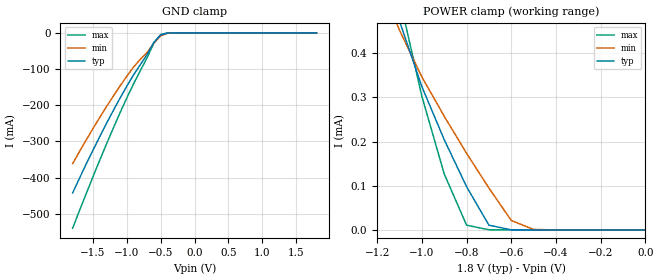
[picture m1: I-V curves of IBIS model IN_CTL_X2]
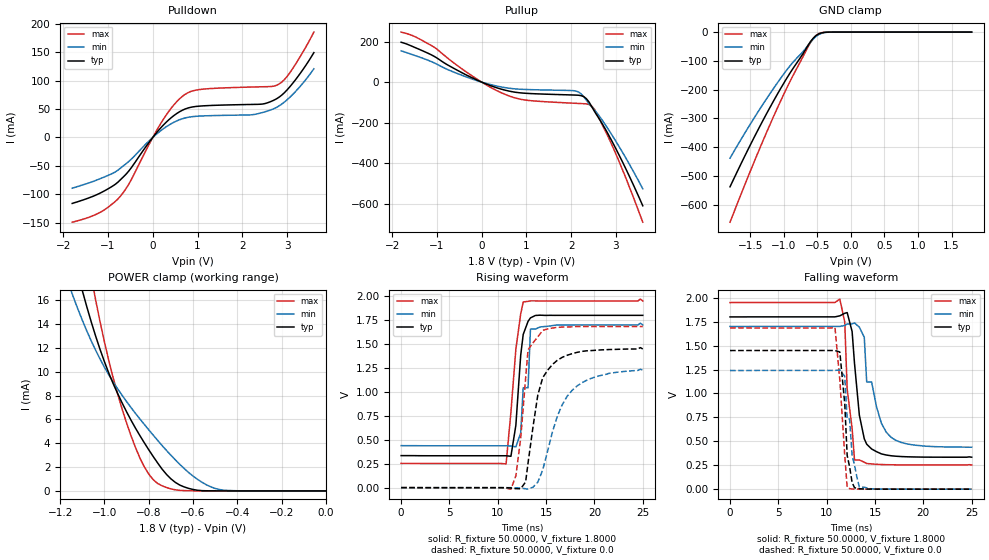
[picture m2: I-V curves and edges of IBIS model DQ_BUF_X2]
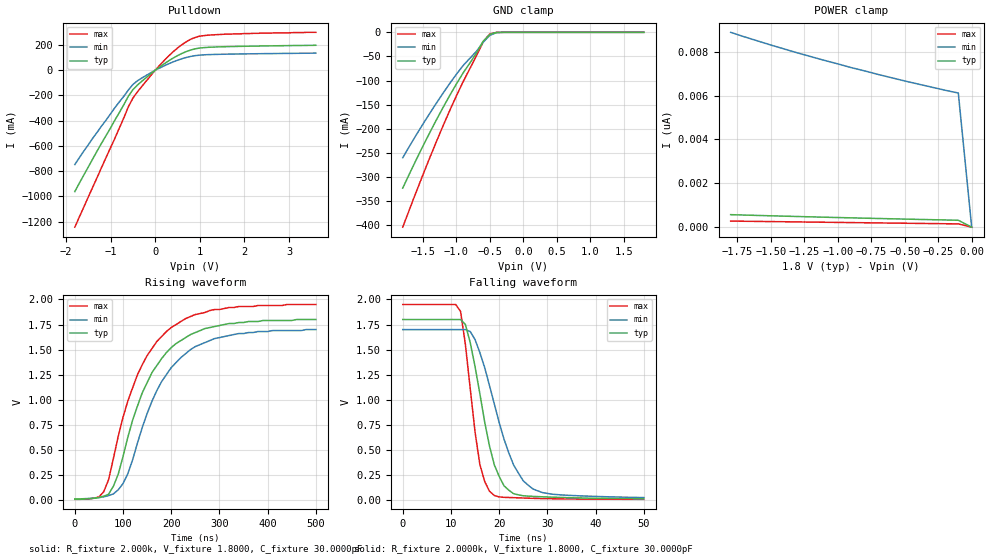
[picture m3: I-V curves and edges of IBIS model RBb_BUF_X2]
| This IBIS file was created by s2ibis3 version 1.1
| North Carolina State University, ERL, 2006
[IBIS ver] 3.2
[File name] s34ms08g2_a_i_18_r2.ibs
[File Rev] 2.0
| Rev1.0 Initial release (X8 LEGACY/ONFI F32 1CE T463ADTX 41086 U785)
| Rev2.0 Update c-comp with measurement
[Date] 1/15/2015
[Source] Cypress IBIS team
[Notes]  Generated IBIS models from SPICE simulations.
|   VIO=1.8V, Temperature Range: Industrial (-40oC to +85oC).
[Disclaimer] THE MODEL LIBRARIES ARE PROVIDED AS IS.
[Copyright] (C) COPYRIGHT 2015
| CYPRESS SEMICONDUCTOR
| ALL RIGHTS RESERVED.
|   Component S34MS08G2 X8 LEGACY/ONFI F32 in VLD063 package
[Component]   S34MS08G2
[Manufacturer]   Cypress
[Package]
| variable   typ   min   max
R_pkg   397.45mOhm   304.71mOhm   533.44mOhm
L_pkg   11.19nH   6.95nH   17.07nH
C_pkg   0.84pF   0.56pF   2.16pF
[Pin]   signal_name   model_name   R_pin   L_pin   C_pin
A1   R   NC
A2   R   NC
A9   R   NC
A10   R   NC
B1   R   NC
B9   R   NC
B10   R   NC
C3   WP   IN_CTL_X2   370.91m   10.638n   2.1652p
C4   ALE   IN_CTL_X2   519.77m   16.877n   0.9751p
C5   VSS   GND
C6   CE#   IN_CTL_X2   533.44m   17.071n   0.9422p
C7   WE#   IN_CTL_X2   393.70m   13.183n   1.0635p
C8   RB#   RBb_BUF_X2  518.54m   16.890n   0.9564p
D3   VCC   NC
D4   RE#   IN_CTL_X2   520.86m   16.856n   0.9647p
D5   CLE   IN_CTL_X2   528.38m   17.047n   0.9436p
D6   R   NC
D7   R   NC
D8   R   NC
E3   R   NC
E4   R   NC
E5   R   NC
E6   R   NC
E7   R   NC
E8   R   NC
F3   R   NC
F4   R   NC
F5   R   NC
F6   R   NC
F7   VSS   NC
F8   R   NC
G3   R   NC
G4   VCC   NC
G5   R   NC
G6   R   NC
G7   R   NC
G8   R   NC
H3   R   NC
H4   IO0   DQ_BUF_X2   310.3m   7.0831n   0.5602p
H5   R   NC
H6   R   NC
H7   R   NC
H8   VCC   POWER
J3   R   NC
J4   IO1   DQ_BUF_X2   313.03m   7.0798n   0.5804p
J5   R   NC
J6   VCC   POWER
J7   IO5   DQ_BUF_X2   330.01m   7.7748n   0.5936p
J8   IO7   DQ_BUF_X2   318.00m   7.1125n   0.5636p
K3   VSS   GND
K4   IO2   DQ_BUF_X2   338.07m   7.8156n   0.5782p
K5   IO3   DQ_BUF_X2   329.94m   7.6927n   0.5743p
K6   IO4   DQ_BUF_X2   331.98m   7.8931n   0.5927p
K7   IO6   DQ_BUF_X2   304.71m   6.9573n   0.5904p
K8   VSS   GND
L1   R   NC
L2   R   NC
L9   R   NC
L10   R   NC
M1   R   NC
M2   R   NC
M9   R   NC
M10   R   NC
| Models and submodels in the file (3): IN_CTL_X2 (Input), DQ_BUF_X2 (I/O), RBb_BUF_X2 (Open_drain)
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|   Model IN_CTL_X2
[Model]   IN_CTL_X2
Model_type   Input
Vinl =   0.3600V
Vinh =   1.4400V
C_comp   6.24pF   5.62pF   8.16pF
[Temperature Range]   25.0000   85.0000   -40.0000
[Voltage Range]   1.8000V   1.7000V   1.9500V
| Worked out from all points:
|   GND clamp passes 1 mA (typ) near -0.41 V on its own axis
|   POWER clamp passes 1 mA (typ) near -1.37 V on its own axis
[GND_clamp]
| voltage   I(typ)   I(min)   I(max)
-1.8V     -442.4mA   -361.4mA   -539.8mA
-1.6V     -362.6mA   -296mA     -444.4mA
-1.4V     -286.6mA   -233.8mA   -351.8mA
-1.1V     -180.2mA   -146.7mA   -220.6mA
-900mV    -115.8mA   -94.34mA   -140.5mA
-700mV    -59.7mA    -54.06mA   -67.86mA
-600mV    -25.92mA   -27.82mA   -28.04mA
-500mV    -5.764mA   -7.906mA   -4.376mA
-400mV    -434.2uA   -908.8uA   -145.6uA
-300mV    -17.2uA    -67.78uA   -1.974nA
1.8V      304.6pA    5.746nA    151.5pA
[POWER_clamp]
| voltage   I(typ)   I(min)   I(max)
-1.8V     2.01mA     1.613mA    2.604mA
-1.1V     472.8uA    452.2uA    525uA
-1V       324.4uA    346.4uA    302.6uA
-900mV    204.4uA    257.4uA    126.8uA
-800mV    97.92uA    173.5uA    10.85uA
-700mV    10.78uA    94.82uA    474.4nA
-600mV    352.6nA    21.46uA    12.99nA
-500mV    11.72nA    1.19uA     416.2pA
0V        0A         0A         0A
|   Model DQ_BUF_X2
[Model]  DQ_BUF_X2
Model_type I/O
Vinl =   0.3600V
Vinh =   1.4400V
Vmeas =  0.9000V
Cref =   30.0000pF
C_comp   7.02pF   6.32pF   9.00pF
[Temperature Range]   25.0000   85.0000   -40.0000
[Pullup Reference]   1.8000V   1.7000V   1.9500V
[Pulldown Reference]   0.0V   0.0V   0.0V
[POWER Clamp Reference]   1.8000V   1.7000V   1.9500V
[GND Clamp Reference]   0.0V   0.0V   0.0V
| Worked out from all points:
|   slope of the pulldown table from 0 to 0.27 V, typ, clamps not added: 11.1 ohm
|   slope of the pullup table from 0 to 0.27 V, typ, clamps not added: 11.7 ohm
|   GND clamp passes 1 mA (typ) near -0.39 V on its own axis
|   POWER clamp passes 1 mA (typ) near -0.70 V on its own axis
|   rising waveform, R_fixture 50.0000, V_fixture 1.8000: 20-80 % time 686ps typ, 859ps min, 915ps max; typ from 0.335 V to 1.8 V
|   rising waveform, R_fixture 50.0000, V_fixture 0.0: 20-80 % time 1.54ns typ, 2.6ns min, 909ps max; typ from 0.001 V to 1.45 V
|   falling waveform, R_fixture 50.0000, V_fixture 1.8000: 20-80 % time 946ps typ, 1.69ns min, 744ps max; typ from 1.8 V to 0.334 V
|   falling waveform, R_fixture 50.0000, V_fixture 0.0: 20-80 % time 635ps typ, 913ps min, 710ps max; typ from 1.45 V to 0 V
[Pulldown]
|Voltage   I(typ)   I(min)   I(max)
-1.8V     -116.2mA   -89.4mA    -149.2mA
-1.2V     -98.95mA   -73.41mA   -132.9mA
-780mV    -78.88mA   -57.77mA   -108.5mA
-540mV    -59.55mA   -42.61mA   -82.78mA
180mV     16.92mA    11.85mA    24.75mA
420mV     35.15mA    24.4mA     52.18mA
660mV     47.71mA    32.75mA    72.06mA
1.08V     55.19mA    37.59mA    84.45mA
2.22V     57.93mA    39.8mA     88.58mA
2.76V     67.57mA    52.52mA    91.45mA
3.06V     88.75mA    70.28mA    113.3mA
3.6V      149.1mA    120.6mA    185.2mA
[Pullup]
|Voltage   I(typ)   I(min)   I(max)
-1.8V     197mA      154.7mA    247.2mA
-1.5V     171.9mA    132.2mA    225.6mA
-1.08V    129.6mA    96.99mA    175mA
-180mV    17.93mA    12.87mA    25.74mA
540mV     -40.6mA    -27.74mA   -61.98mA
1.02V     -55.58mA   -36.59mA   -89.75mA
2.1V      -63.96mA   -43.71mA   -104.6mA
2.28V     -71.41mA   -71.84mA   -106.5mA
2.46V     -121.1mA   -122.7mA   -118.4mA
2.58V     -165.4mA   -153.5mA   -157.5mA
2.94V     -303.8mA   -271.2mA   -324.9mA
3.6V      -610.8mA   -527mA     -691.8mA
[GND_clamp]
|Voltage   I(typ)   I(min)   I(max)
-1.8V     -538mA     -438.4mA   -661.2mA
-1.44V    -365.9mA   -298.5mA   -451mA
-1.24V    -277.1mA   -226.4mA   -340.6mA
-1.08V    -210mA     -171.9mA   -256.7mA
-880mV    -133mA     -110mA     -159.6mA
-720mV    -77.76mA   -69.99mA   -88.72mA
-640mV    -46.97mA   -46.75mA   -52.06mA
-560mV    -21.24mA   -24.35mA   -22.11mA
-520mV    -12.43mA   -15.31mA   -11.88mA
-440mV    -3.106mA   -4.606mA   -2.241mA
-320mV    -145.2uA   -332.9uA   -46.3uA
1.8V      457.2pA    18.09nA    -155pA
[POWER_clamp]
|Voltage   I(typ)   I(min)   I(max)
-1.8V     89.64mA    69.3mA     119.4mA
-1.14V    19.73mA    16.27mA    26.61mA
-1.1V     16.83mA    14.34mA    22.17mA
-1.06V    14.22mA    12.61mA    18.02mA
-1.04V    13.02mA    11.82mA    16.06mA
-960mV    8.984mA    9.13mA     9.456mA
-880mV    5.94mA     6.999mA    4.631mA
-820mV    4.042mA    5.586mA    2.019mA
-760mV    2.352mA    4.25mA     626.6uA
-660mV    492uA      2.236mA    46.59uA
-500mV    4.728uA    208uA      481.5nA
0V        457.2pA    8.03nA     254.7pA
[Ramp]
| variable   typ   min   max
dV/dt_r  0.8687/1.5076n   0.7357/2.5719n   1.0099/0.9060n
dV/dt_f  0.8792/0.9315n   0.7565/1.6135n   1.0178/0.5697n
R_load = 50.0000
[Rising Waveform]
R_fixture= 50.0000
V_fixture= 1.8000
V_fixture_min= 1.7000
V_fixture_max= 1.9500
|time   V(typ)   V(min)   V(max)
0s        334.9mV    439mV      253.7mV
10.86ns   333.3mV    437.8mV    247.8mV
11.36ns   328.1mV    435mV      789.7mV
11.87ns   652.1mV    426.7mV    1.447V
12.37ns   1.382V     570.5mV    1.814V
12.63ns   1.601V     1.043V     1.94V
13.13ns   1.737V     1.043V     1.946V
13.38ns   1.773V     1.656V     1.951V
16.41ns   1.8V       1.7V       1.95V
25ns      1.8V       1.7V       1.95V
[Rising Waveform]
R_fixture= 50.0000
V_fixture= 0.0
V_fixture_min= 0.0
V_fixture_max= 0.0
|time   V(typ)   V(min)   V(max)
0s        684.5uV    752.3uV    544.4uV
11.36ns   -3.473mV   193uV      -15.25mV
11.87ns   -10.1mV    -1.106mV   123.5mV
12.37ns   -11.06mV   -4.621mV   515.8mV
13.13ns   256.6mV    -15.53mV   1.44V
14.14ns   967.3mV    57.91mV    1.576V
14.65ns   1.149V     185.6mV    1.643V
16.16ns   1.331V     746.9mV    1.674V
17.68ns   1.399V     1.016V     1.68V
25ns      1.448V     1.227V     1.684V
[Falling Waveform]
R_fixture= 50.0000
V_fixture= 1.8000
V_fixture_min= 1.7000
V_fixture_max= 1.9500
|time   V(typ)   V(min)   V(max)
0s        1.799V     1.699V     1.95V
11.36ns   1.811V     1.7V       1.986V
11.87ns   1.837V     1.71V      1.745V
12.12ns   1.845V     1.726V     1.045V
12.63ns   1.647V     1.726V     635.1mV
12.88ns   1.313V     1.737V     305.2mV
13.89ns   526.1mV    1.586V     281.7mV
14.14ns   469.8mV    1.12V      268mV
16.16ns   356.9mV    595.5mV    255.8mV
25ns      334mV      438.5mV    253.2mV
[Falling Waveform]
R_fixture= 50.0000
V_fixture= 0.0
V_fixture_min= 0.0
V_fixture_max= 0.0
|time   V(typ)   V(min)   V(max)
0s        1.448V     1.239V     1.685V
10.86ns   1.448V     1.24V      1.688V
11.36ns   1.433V     1.246V     1.141V
11.87ns   891.6mV    1.179V     351.2mV
12.12ns   351.8mV    732.3mV    19.33mV
12.37ns   234.9mV    732.3mV    5.699mV
12.63ns   70.13mV    353.3mV    1.888mV
12.88ns   15.28mV    251.7mV    886.1uV
13.38ns   4.126mV    20.97mV    442.6uV
25ns      -10.09uV   -12.98uV   4.692uV
|   Model RBb_BUF_X2
[Model]   RBb_BUF_X2
Model_type   Open_drain
Polarity   Non-Inverting
Enable   Active-High
Vmeas =   0.9000V
Cref =  30.0000pF
Rref =   2.0000k
Vref =   1.8000V
C_comp   7.76pF   6.98pF   9.12pF
[Temperature Range]   25.0000   85.0000   -40.0000
[Voltage Range]   1.8000V   1.7000V   1.9500V
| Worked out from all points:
|   slope of the pulldown table from 0 to 0.27 V, typ, clamps not added: 4.06 ohm
|   GND clamp passes 1 mA (typ) near -0.42 V on its own axis
|   rising waveform, R_fixture 2.000k, V_fixture 1.8000, C_fixture 30.0000pF: 20-80 % time 89ns typ, 92.2ns min, 88.1ns max; typ from 0.007 V to 1.8 V
|   falling waveform, R_fixture 2.0000k, V_fixture 1.8000, C_fixture 30.0000pF: 20-80 % time 4.36ns typ, 6.21ns min, 2.91ns max; typ from 1.8 V to 0.013 V
[Pulldown]
| voltage   I(typ)   I(min)   I(max)
-1.8V     -962mA     -748mA     -1.244A
-1.2V     -578mA     -442mA     -770mA
-900mV    -394mA     -296mA     -538mA
-600mV    -206mA     -156.6mA   -290mA
-500mV    -155mA     -113.8mA   -222mA
0V        0A         0A         0A
300mV     73.6mA     50.4mA     112mA
500mV     115.2mA    78.8mA     175.4mA
800mV     160.4mA    109.2mA    246mA
1V        175.6mA    119.2mA    270mA
1.6V      186.4mA    126.8mA    286mA
3.6V      197.4mA    135.2mA    300mA
[POWER_clamp]
| voltage   I(typ)   I(min)   I(max)
-1.8V     570pA      8.89nA     277pA
-1.3V     486pA      7.95nA     239pA
-900mV    425pA      7.28nA     209pA
-500mV    368pA      6.67nA     179pA
-100mV    315pA      6.12nA     149pA
0V        0A         0A         0A
[GND_clamp]
| voltage   I(typ)   I(min)   I(max)
-1.8V     -322.6mA   -259.7mA   -403.5mA
-1.6V     -264.2mA   -212.9mA   -331mA
-1.4V     -208.7mA   -168.5mA   -261mA
-1.1V     -131.2mA   -106.3mA   -162.5mA
-900mV    -84.49mA   -69.13mA   -102.8mA
-700mV    -43.04mA   -39.48mA   -48.7mA
-600mV    -18.71mA   -20.67mA   -20.21mA
-500mV    -4.313mA   -6.267mA   -3.275mA
-400mV    -343uA     -738.6uA   -116.7uA
-300mV    -13.93uA   -55.22uA   -1.645uA
1.8V      302.1pA    6.118nA    134pA
[Ramp]
| variable   typ   min   max
dV/dt_r   1.08/29n   1.02/37.6n   1.17/22.3n
dV/dt_f   1.08/0.759n   1.02/1.19n   1.17/0.463n
R_load = 50.0000
[Rising Waveform]
R_fixture = 2.000k
V_fixture = 1.8000
V_fixture_min = 1.7000
V_fixture_max = 1.9500
C_fixture = 30.0000pF
| time   V(typ)   V(min)   V(max)
0s        6.56mV     8.95mV     4.73mV
60ns      36.1mV     29.4mV     80.9mV
80ns      136mV      59.1mV     412mV
100ns     433mV      162mV      825mV
140ns     1.07V      724mV      1.35V
170ns     1.34V      1.09V      1.58V
200ns     1.52V      1.32V      1.72V
240ns     1.65V      1.5V       1.83V
290ns     1.73V      1.61V      1.9V
500ns     1.8V       1.7V       1.95V
[Falling Waveform]
R_fixture = 2.0000k
V_fixture = 1.8000
V_fixture_min = 1.7000
V_fixture_max = 1.9500
C_fixture = 30.0000pF
| time   V(typ)   V(min)   V(max)
0s        1.8V       1.7V       1.95V
12ns      1.8V       1.7V       1.88V
13ns      1.75V      1.7V       1.55V
14ns      1.57V      1.68V      1.11V
16ns      1.06V      1.47V      354mV
17ns      777mV      1.32V      184mV
19ns      350mV      957mV      44.4mV
23ns      63mV       349mV      23.4mV
27ns      35.9mV     110mV      16.7mV
50ns      12.6mV     24.4mV     6.75mV
